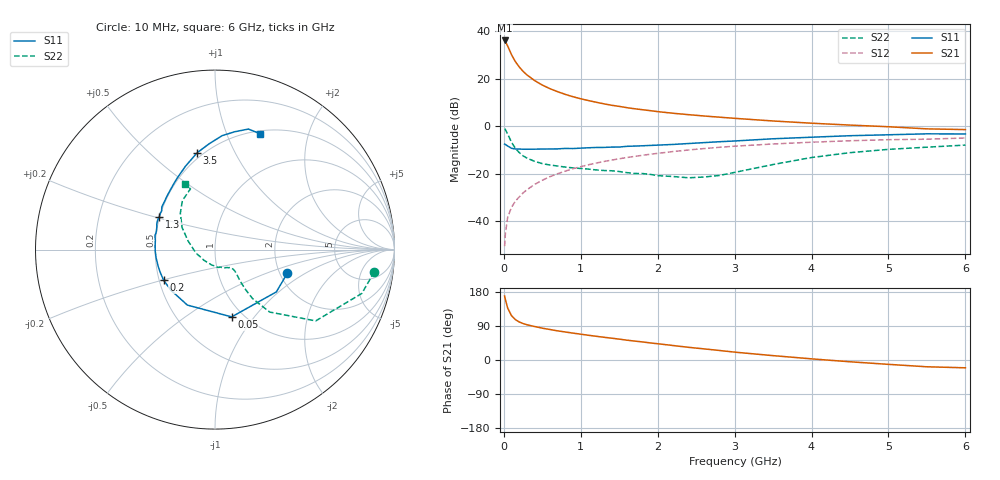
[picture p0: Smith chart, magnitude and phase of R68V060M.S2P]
! SIEMENS Small Signal Semiconductors
! BFR193
! Si NPN RF Bipolar Junction Transistor in SOT23
! VCE = 8 V  IC = 60 mA
! Common Emitter S-Parameters:  May  1996
# GHz  S  MA  R  50
!  f  S11  S21  S12  S22
! GHz  MAG  ANG  MAG  ANG  MAG  ANG  MAG  ANG
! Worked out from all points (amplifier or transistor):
!   36 points, 10 MHz to 6 GHz, reference 50 ohm
!   highest |S21| = 36.2 dB at 10 MHz (marker M1)
!   |S21| within 3 dB of that: start of sweep to 58.9 MHz
!   unconditionally stable (mu >= 1): 410.8 MHz to 2.165 GHz
!   at 250 MHz: K = 0.94, MSG = 25.6 dB, |S12| = -28.0 dB
!   at 1.4 GHz: K = 1.02, MAG = 10.6 dB, |S12| = -14.2 dB
!   at 6 GHz: K = 0.95, MSG = 1.8 dB, |S12| = -4.9 dB
!   S11 on the Smith chart (normalised r, x): 10 MHz: 2.20, -0.70; 50 MHz: 0.88, -0.78; 200 MHz: 0.53, -0.20; 1.3 GHz: 0.50, +0.21; 3.5 GHz: 0.47, +0.72; 6 GHz: 0.53, +1.32
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0.01  0.4242 -18.0  64.55 169.1  0.003 79.3  0.8957 -8.0
0.02  0.4151 -34.6  61.58 159.4  0.0055 77.8  0.854 -16.6
0.05  0.3862 -76.1  49.25 137.0  0.0122 68.7  0.6875 -35.3
0.1  0.3453 -116.5  32.34 116.9  0.0198 67.2  0.4625 -48.8
0.15  0.3339 -137.1  23.11 106.5  0.0266 68.2  0.3452 -52.5
0.2  0.3333 -149.4  17.89 100.4  0.0327 70.6  0.2809 -52.6
0.25  0.3304 -157.8  14.45 96.2  0.0397 71.4  0.2394 -51.8
0.3  0.3301 -163.3  12.15 93.0  0.0462 72.7  0.215 -50.8
0.4  0.3314 -172.4  9.237 88.3  0.0599 73.4  0.1837 -48.7
0.5  0.3332 -178.7  7.411 84.0  0.0733 73.7  0.1644 -47.3
0.6  0.3345 175.5  6.221 80.4  0.0874 72.8  0.1536 -47.0
0.7  0.336 171.4  5.372 76.9  0.1009 72.1  0.1461 -47.4
0.8  0.3433 166.9  4.716 73.9  0.1145 70.8  0.1389 -48.1
0.9  0.3416 163.1  4.211 70.9  0.1286 69.9  0.1335 -48.7
1.1  0.3544 156.3  3.499 65.3  0.1555 67.5  0.1261 -53.3
1.3  0.3606 149.5  2.989 60.0  0.1822 64.8  0.1177 -58.2
1.7  0.3849 138.4  2.351 50.0  0.2333 59.0  0.1018 -72.9
2.2  0.4166 126.4  1.891 38.2  0.2951 51.6  0.0879 -102.2
3.5  0.5484 100.5  1.3 11.5  0.4263 31.5  0.1575 162.2
4.5  0.6362 86.4  1.065 -4.7  0.4986 17.6  0.2796 133.7
5.5  0.697 74.5  0.887 -17.9  0.5372 4.1  0.3649 112.0
6  0.6925 68.9  0.856 -20.6  0.5703 0.2  0.4039 114.3
